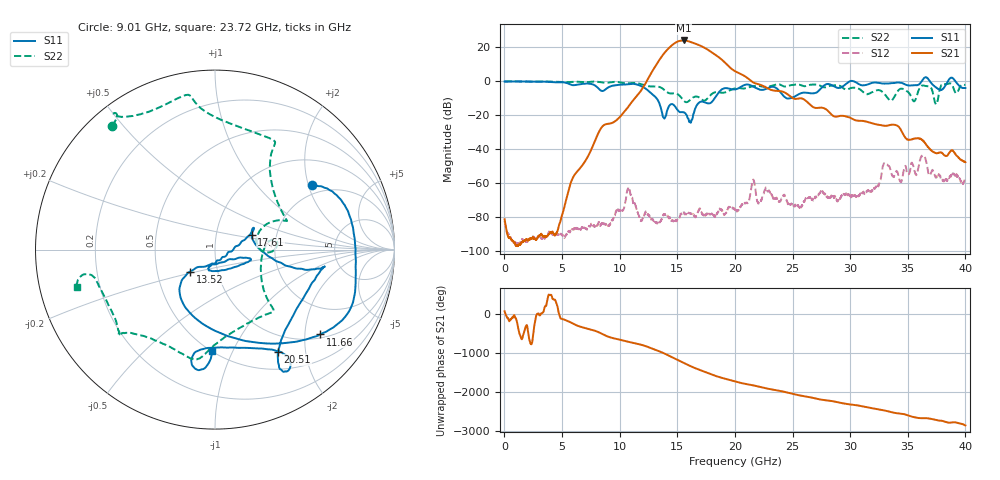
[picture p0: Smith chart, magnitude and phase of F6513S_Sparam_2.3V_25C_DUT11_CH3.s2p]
!Keysight Technologies,N5245B,MY57181321,A.14.80.03
!Date: Thursday, January 06, 2022 14:49:54
!Correction: S11(C  2-Port  )
!S21(C  2-Port  )
!S12(C  2-Port  )
!S22(C  2-Port  )
!S2P File: Measurements: S11, S21, S12, S22:
# Hz S  dB  R 50
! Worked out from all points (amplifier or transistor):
!   4000 points, 10 MHz to 40 GHz, reference 50 ohm
!   highest |S21| = 23.9 dB at 15.54 GHz (marker M1)
!   |S21| within 3 dB of that: 14.5 GHz to 16.97 GHz (2.467 GHz wide, 15.7 % of centre)
!   unconditionally stable (mu >= 1): start of sweep to 30.03 GHz; 30.22 GHz to 36.23 GHz; 36.91 GHz to 38.49 GHz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
!   at 6.67 GHz: K = 157013.32, MAG = -36.9 dB, |S12| = -86.6 dB
!   at 20.01 GHz: K = 694.71, MAG = 9.4 dB, |S12| = -75.9 dB
!   at 40 GHz: K = 21603.89, MAG = -42.0 dB, |S12| = -56.6 dB
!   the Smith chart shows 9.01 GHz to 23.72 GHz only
!   S11 on the Smith chart (normalised r, x): 9.01 GHz: 1.71, +2.12; 11.66 GHz: 1.10, -2.39; 13.52 GHz: 0.74, -0.19; 17.61 GHz: 1.48, +0.26; 20.51 GHz: 0.74, -1.53; 23.72 GHz: 0.50, -0.84
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1e7  -0.29 179.0  -81.57 72.3  -82.55 -53.4  -0.29 -179.9
6.68e9  -1.80 64.5  -50.41 29.5  -86.50 -85.2  -0.61 154.1
9.01e9  -3.76 33.4  -25.24 141.5  -85.22 -14.8  -0.93 129.7
1.166e10  -2.47 -38.9  -7.40 -48.4  -79.55 -42.3  -1.49 98.2
1.334e10  -11.70 -136.4  11.39 139.3  -83.59 24.9  -3.34 60.6
1.352e10  -14.64 -138.6  13.22 118.3  -82.99 -63.9  -3.71 60.2
1.406e10  -19.10 -29.1  17.97 46.9  -78.88 35.0  -6.32 48.9
1.456e10  -13.62 -16.8  21.23 -26.0  -82.49 -74.8  -7.33 24.9
1.506e10  -17.49 -52.6  23.35 -98.6  -81.34 21.0  -7.94 24.1
1.554e10  -18.38 -106.1  23.91 -168.2  -76.95 14.9  -11.50 22.2
1.594e10  -22.07 -99.0  23.49 136.2  -78.51 168.3  -12.13 1.4
1.627e10  -22.81 -16.5  22.72 91.9  -78.37 121.2  -10.20 -2.6
1.689e10  -12.69 25.3  21.15 17.3  -75.89 134.3  -9.72 9.9
1.761e10  -13.14 22.3  18.62 -64.0  -78.81 57.5  -10.34 -31.7
1.846e10  -8.02 -12.5  14.69 -155.3  -78.08 73.8  -6.50 -47.0
1.913e10  -4.21 -9.0  10.87 147.0  -78.62 -23.8  -6.81 -72.3
2.001e10  -5.01 -35.8  5.76 74.9  -75.90 -6.9  -4.34 -97.6
2.051e10  -3.49 -58.3  4.11 37.9  -73.97 -167.7  -4.30 -106.9
2.372e10  -4.92 -91.5  -5.86 -155.6  -70.03 -136.4  -1.97 -164.8
2.667e10  -7.35 -69.5  -14.87 22.4  -69.37 171.4  -2.14 151.0
3.334e10  -1.45 -165.1  -26.14 26.8  -50.11 33.4  -10.72 152.3
4e10  -4.15 82.6  -47.90 29.7  -56.64 157.5  -2.34 160.7
